(* Logix 5000 DataType export Banner_ISD_Dual_Chain_Status_v1; software revision 32.00 *)

TYPE Banner_Chain_Status_v1 :
STRUCT
   Device_Count_Mismatch : BOOL;   // 0 = False, 1 = True
   Device_Order_Mismatch : BOOL;   // 0 = False, 1 = True
   No_Diagnostics_Data_Detected : BOOL;   // 0 = False, 1 = True
   bit3 : BOOL;
   Incompatible_Device : BOOL;   // 0 = False, 1 = True
   ISD_Terminator_Missing : BOOL;   // 0 = False, 1 = True
   ISD_Actuator_Not_Taught : BOOL;   // 0 = False, 1 = True
   ISD_Wrong_Actuator : BOOL;   // 0 = False, 1 = True
   ISD_Internal_Error : BOOL;   // 0 = False, 1 = True
   ISD_Output_Fault_Detected : BOOL;   // 0 = False, 1 = True
   ISD_Chain_Change_Detected : BOOL;   // 0 = False, 1 = True
   bit11 : BOOL;
   ISD_OSSD_Status : BOOL;   // 0 = Off, 1 = ON
   bit13 : BOOL;
   bit14 : BOOL;
   bit15 : BOOL;
   bit16 : BOOL;
   bit17 : BOOL;
   bit18 : BOOL;
   bit19 : BOOL;
   bit20 : BOOL;
   bit21 : BOOL;
   bit22 : BOOL;
   bit23 : BOOL;
   bit24 : BOOL;
   bit25 : BOOL;
   bit26 : BOOL;
   bit27 : BOOL;
   bit28 : BOOL;
   bit29 : BOOL;
   bit30 : BOOL;
   bit31 : BOOL;
END_STRUCT
END_TYPE

TYPE Banner_ISD_Dual_Chain_Status_v1 :   // UDT that gives the overall Chain information for an ISD device.
STRUCT
   C1_Inputs : DINT;
   C2_Inputs : DINT;
   C1_On_Off : DINT;
   C2_On_Off : DINT;
   C1_Fault : DINT;
   C2_Fault : DINT;
   C1_Marginal : DINT;
   C2_Marginal : DINT;
   C1_Alert : DINT;
   C2_Alert : DINT;
   C1_Reset : DINT;
   C2_Reset : DINT;
   C1_Actuator_State : DINT;
   C2_Actuator_State : DINT;
   C1_Series_Status : Banner_Chain_Status_v1;
   C2_Series_Status : Banner_Chain_Status_v1;
END_STRUCT
END_TYPE
